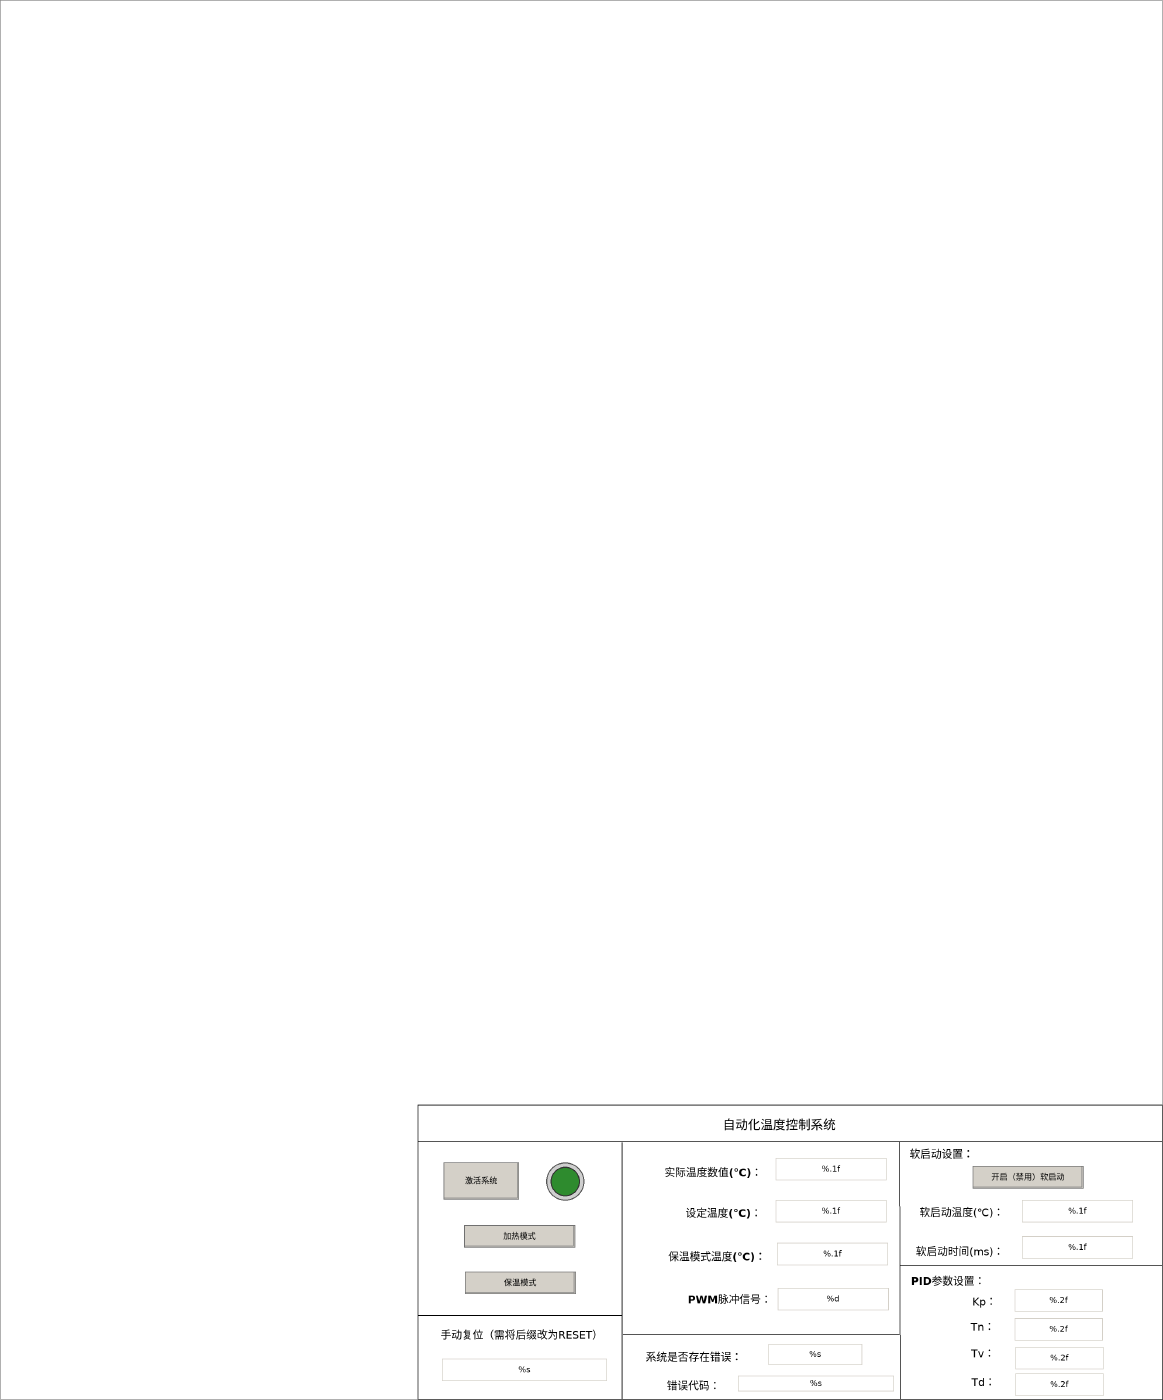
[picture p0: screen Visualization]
VISUALIZATION Visualization  // 1576x1897
    Rectangle (566,1497 1010x400)
    Line (1576,1547) (567,1547)
    Label (910,1502 292x44), "自动化温度控制系统"
    Button (601,1575 102x50), "激活系统"
        toggle MAIN.bStart p2164770859=TRUE
    Line (843,1897) (843,1548)
    Lamp1 (736,1570 60x62), variable: MAIN.bStart, style: Lamp-Lamp1-Green
    Button (629,1660 150x30), "加热模式"
        toggle Controller_v2.bSelSetpoint p2164770859=TRUE
    Button (630,1723 150x30), "保温模式"
        toggle Controller_v2.bSelSetpoint p2164770859=TRUE
    Textfield (1051,1569 150x30), "%.1f", text variable: Controller_v2.ftemp
    Textfield (1051,1626 150x30), "%.1f", text variable: Controller_v2.fW1
        OnMouseClick: write the text variable via Default
    Textfield (1053,1684 150x30), "%.1f", text variable: Controller_v2.fW2
        OnMouseClick: write the text variable via Default
    Textfield (1054,1745 150x30), "%d", text variable: Controller_v2.bYPWMPos
    Label (891,1570 151x38), "实际温度数值(℃)："
    Label (917,1626 127x36), "设定温度(℃)："
    Label (898,1685 147x36), "保温模式温度(℃)："
    Label (929,1743 120x36), "PWM脉冲信号："
    Line (1218,1808) (844,1808)
    Label (858,1826 165x26), "系统是否存在错误："
    Label (865,1863 150x30), "错误代码："
    Textfield (1000,1864 211x21), "%s", text variable: Controller_v2.eErrorId
    Textfield (1041,1821 127x28), "%s", text variable: Controller_v2.bError
    Textfield (599,1841 223x30), "%s", text variable: Controller_v2.eCTRL_Mode
        OnMouseClick: write the text variable via Default
    Label (579,1796 256x26), "手动复位（需将后缀改为RESET）"
    Line (567,1782) (842,1782)
    Line (1234,1549)
    Line (1220,1896) (1219,1547)
    Button (1318,1580 150x30), "开启（禁用）软启动"
        toggle Controller_v2.stControllerParameter.bEnableSoftStart p2164770859=TRUE
    Line (1575,1715) (1220,1715)
    Label (1213,1546 126x36), "软启动设置："
    Label (1235,1625 137x36), "软启动温度(℃)："
    Label (1231,1678 140x36), "软启动时间(ms)："
    Textfield (1385,1626 150x30), "%.1f", text variable: Controller_v2.stControllerParameter.fWStartUp
        OnMouseClick: write the text variable via Default
    Textfield (1385,1675 150x30), "%.1f", text variable: Controller_v2.stControllerParameter.tStartUp
        OnMouseClick: write the text variable via Default
    Label (1222,1718 126x36), "PID参数设置："
    Label (1271,1746 126x36), "Kp："
    Label (1269,1780 126x36), "Tn："
    Label (1269,1816 126x36), "Tv："
    Label (1270,1855 126x36), "Td："
    Textfield (1375,1747 119x30), "%.2f", text variable: Controller_v2.stControllerParameter.fTuneKp
        OnMouseClick: write the text variable via Default
    Textfield (1375,1786 119x30), "%.2f", text variable: Controller_v2.stControllerParameter.fTuneTn
        OnMouseClick: write the text variable via Default
    Textfield (1376,1825 119x30), "%.2f", text variable: Controller_v2.stControllerParameter.fTuneTv
        OnMouseClick: write the text variable via Default
    Textfield (1376,1861 119x30), "%.2f", text variable: Controller_v2.stControllerParameter.fTuneTd
        OnMouseClick: write the text variable via Default
END_VISUALIZATION
